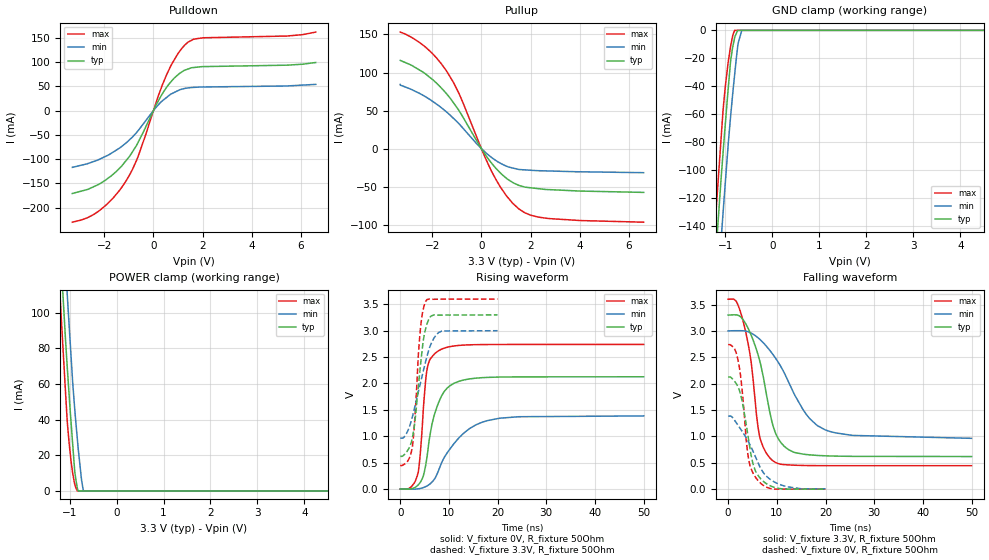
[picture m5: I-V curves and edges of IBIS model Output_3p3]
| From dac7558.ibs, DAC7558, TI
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|   TRISTATE OUTPUT 3.3V Model
[Model]   Output_3p3
Model_type   3-state
Polarity   Non-Inverting
Enable   Active-High
Vmeas = 1.65
Vref = 1.65
Cref = 15pF
Rref = 50
|   typ   min   max
|   (nom PVT)   (fast PVT)  (slow PVT)
|Average
C_comp   8.687e-12   7.507e-12   1.038e-11
|ON state : BUFFER OUTPUT TURNED HIGH
|C_comp   1.626e-11   1.392e-11   1.962e-11
|OFF state: BUFFER in HIGH IMPEDANCE for IOs and 3-state,
|This is BUFFER in LOW state for OUTPUT only type
|C_comp   1.110e-12   1.097e-12   1.131e-12
|Where  nom PVT is Nominal Process, 3.3V, 25C
|   fast PVT is Strong Process, 3.6V, -40C
|   slow PVT is Weak Process, 3.0V, 105C
[Voltage Range]   3.3   3   3.6
|Ambient Temperature   25   105   -40
|Junction Temperature
[Temperature Range]   25   105   -40
[Pullup Reference]   3.3   3   3.6
[Pulldown Reference]   0   0   0
[Power Clamp Reference]   3.3   3   3.6
[GND Clamp Reference]   0   0   0
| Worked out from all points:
|   slope of the pulldown table from 0 to 0.495 V, typ, clamps not added: 11 ohm
|   slope of the pullup table from 0 to 0.495 V, typ, clamps not added: 22.3 ohm
|   GND clamp passes 1 mA (typ) near -0.75 V on its own axis
|   POWER clamp passes 1 mA (typ) near -0.83 V on its own axis
|   falling waveform, V_fixture 3.3V, R_fixture 50Ohm: 20-80 % time 4.01ns typ, 7.58ns min, 2.69ns max; typ from 3.3 V to 0.619 V
|   rising waveform, V_fixture 0V, R_fixture 50Ohm: 20-80 % time 3ns typ, 6.19ns min, 1.39ns max; typ from 0 V to 2.13 V
|   rising waveform, V_fixture 3.3V, R_fixture 50Ohm: 20-80 % time 1.83ns typ, 3.23ns min, 1.29ns max; typ from 0.619 V to 3.3 V
|   falling waveform, V_fixture 0V, R_fixture 50Ohm: 20-80 % time 2.51ns typ, 4.72ns min, 1.75ns max; typ from 2.13 V to 0 V
[Pulldown]
|   Voltage   I(typ)   I(min)   I(max)
-3.3V     -170.9mA   -117mA     -230mA
-2.191V   -151.2mA   -100.3mA   -205.8mA
-1.637V   -131.1mA   -85.56mA   -180mA
-1.151V   -105.5mA   -68.28mA   -147.8mA
-625.2mV  -65.56mA   -41.5mA    -94.68mA
188.4mV   18.95mA    11.27mA    29.01mA
541.2mV   48.37mA    27.26mA    74.47mA
969.6mV   72.5mA     40.3mA     115.1mA
1.394V    85.34mA    46.58mA    140.5mA
2.017V    90.47mA    48.47mA    149.8mA
5.437V    93.47mA    50.62mA    153.5mA
6.6V      98.96mA    53.87mA    161.6mA
[GND Clamp]
|   Voltage   I(typ)   I(min)   I(max)
-3.3V     -1.272A    -1.283A    -1.279A
-1.284V   -199.3mA   -241.3mA   -172.4mA
-1.19V    -153.8mA   -196.5mA   -125mA
-1.148V   -133.3mA   -176.3mA   -104.8mA
-1.089V   -105mA     -148.5mA   -76.08mA
-1.05V    -87.7mA    -130.6mA   -57.26mA
-945.6mV  -43.94mA   -83.99mA   -24.15mA
-891mV    -22.57mA   -62.31mA   -11.76mA
-801.9mV  -5.162mA   -31.37mA   0A
-735mV    -216.6uA   -10.61mA   0A
-650.4mV  0A         0A         0A
6.6V      0A         0A         0A
[Pullup]
|   Voltage   I(typ)   I(min)   I(max)
-3.3V     115.9mA    84.24mA    153.1mA
-2.274V   98.17mA    68.19mA    133.4mA
-1.835V   86.37mA    58.73mA    119.5mA
-1.428V   72.43mA    48.51mA    102.5mA
-888mV    48.81mA    31.93mA    70.82mA
0V        0A         0A         0A
487.2mV   -21.87mA   -13.33mA   -34.28mA
1.002V    -38.43mA   -22.83mA   -61.29mA
1.52V     -48.21mA   -27.36mA   -79.05mA
2.014V    -51.44mA   -28.41mA   -87.52mA
2.752V    -53.83mA   -29.34mA   -91.84mA
6.6V      -57.49mA   -31.58mA   -96.61mA
[POWER Clamp]
|   Voltage   I(typ)   I(min)   I(max)
-3.3V     1.239A     1.254A     1.241A
-1.244V   159.3mA    200mA      129.8mA
-1.175V   126.1mA    167.4mA    96.66mA
-1.151V   114.9mA    156.1mA    85.25mA
-1.131V   105.7mA    146.8mA    76.16mA
-1.046V   68.48mA    109.1mA    38.11mA
-970.8mV  39.53mA    76.77mA    17.36mA
-891mV    11.38mA    46.32mA    3.916mA
-834.9mV  1.67mA     29.36mA    0A
-744mV    0A         6.109mA    0A
-700.8mV  0A         0A         0A
6.6V      0A         0A         0A
[Ramp]
R_load = 50
|   typ   min   max
dV/dt_r   1.2759/2.98565e-09   0.828997/6.11506e-09   1.64376/1.38838e-09
dV/dt_f   1.60824/3.99261e-09   1.20631/7.43438e-09   1.89335/2.68024e-09
[Falling Waveform]
V_fixture = 3.3V
V_fixture_min = 3V
V_fixture_max = 3.6V
R_fixture = 50Ohm
C_fixture = 0F
|   Time   V(typ)   V(min)   V(max)
0s        3.3V       3V         3.6V
2.275ns   3.286V     3.003V     3.429V
3.625ns   3.132V     2.996V     2.972V
4.775ns   2.909V     2.956V     2.37V
6.425ns   2.454V     2.846V     1.021V
9.325ns   1.168V     2.537V     529.2mV
12.4ns    749.3mV    2.032V     459.5mV
16ns      657.3mV    1.425V     448.3mV
20ns      632mV      1.121V     445.3mV
50ns      618.6mV    963.4mV    444.4mV
[Rising Waveform]
V_fixture = 0V
V_fixture_min = 0V
V_fixture_max = 0V
R_fixture = 50Ohm
C_fixture = 0F
|   Time   V(typ)   V(min)   V(max)
0s        690.9pV    970.4pV    530.5pV
2.25ns    1.803mV    -3.154mV   40.08mV
3.675ns   76.12mV    2.838mV    305.9mV
4.725ns   243.9mV    25.64mV    1.491V
5.5ns     607.6mV    57.87mV    2.263V
6.525ns   1.23V      130.6mV    2.507V
7.9ns     1.643V     356.5mV    2.622V
12.25ns   2.047V     988.1mV    2.723V
17.82ns   2.115V     1.294V     2.738V
50ns      2.127V     1.385V     2.74V
[Rising Waveform]
V_fixture = 3.3V
V_fixture_min = 3V
V_fixture_max = 3.6V
R_fixture = 50Ohm
C_fixture = 0F
|   Time   V(typ)   V(min)   V(max)
0s        618.6mV    963.4mV    444.4mV
1.575ns   737.9mV    1.107V     535.8mV
2.475ns   964mV      1.362V     785.7mV
2.95ns    1.236V     1.54V      1.27V
3.7ns     1.919V     1.832V     2.513V
4.15ns    2.34V      2.009V     3.038V
5.375ns   3.089V     2.473V     3.578V
6.85ns    3.299V     2.848V     3.596V
8.5ns     3.296V     2.991V     3.598V
20ns      3.3V       3V         3.6V
[Falling Waveform]
|Gnd
V_fixture = 0V
V_fixture_min = 0V
V_fixture_max = 0V
R_fixture = 50Ohm
C_fixture = 0F
|   Time   V(typ)   V(min)   V(max)
0s        2.127V     1.385V     2.74V
1.25ns    2.051V     1.315V     2.672V
2.025ns   1.938V     1.211V     2.445V
2.75ns    1.717V     1.112V     1.988V
3.675ns   1.244V     979.1mV    962.5mV
4.1ns     995.2mV    910mV      628mV
5.575ns   351.1mV    621.1mV    230.8mV
7.25ns    146mV      310.6mV    70.72mV
9.85ns    25.07mV    119mV      854.3uV
20ns      6.055uV    6.523mV    337.8nV
